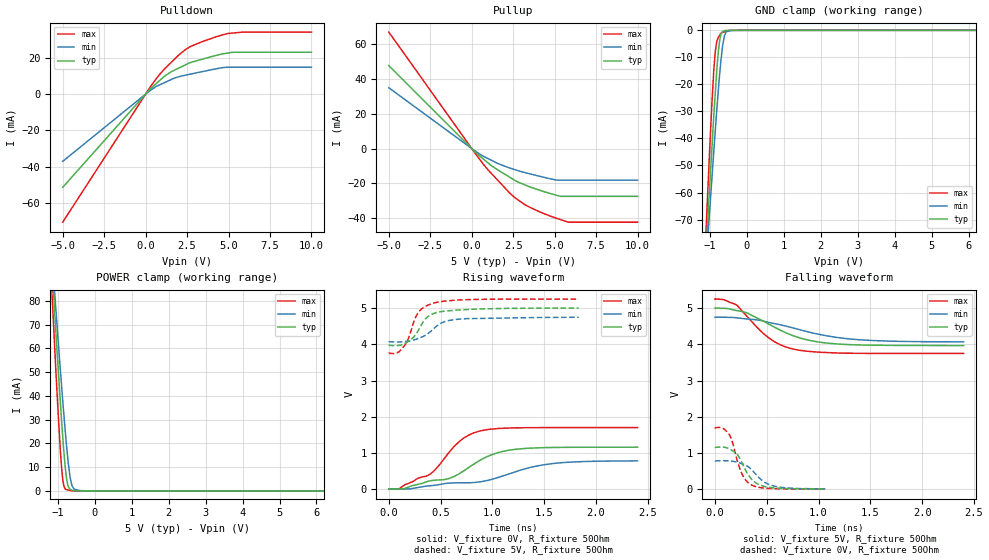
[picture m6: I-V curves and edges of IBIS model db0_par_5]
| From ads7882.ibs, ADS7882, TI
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|   db0_par_5 Model
[Model]   db0_par_5
Model_type   3-state
Polarity   Non-Inverting
Enable   Active-Low
Vmeas = 2.5
Vref = 2.5
Cref = 20pF
Rref = 50
|   typ   min   max
|   (nom PVT)   (Fast PVT)   (slow PVT)
|C_comp from frequency sweep method (F=1.5MHz)
|Average
C_comp   1.566e-12   1.438e-12   1.699e-12
|ON state : BUFFER OUTPUT TURNED HIGH
|C_comp   1.532e-12   1.413e-12   1.655e-12
|OFF state: BUFFER IN HIGH IMPEDANCE
|C_comp   1.600e-12   1.463e-12   1.743e-12
|C_comp from LC tank measurement(L=1nH)
|Resonant Frequency(Hz)   4.580e+09   4.690e+09   4.450e+09
|C_comp   1.209e-12   1.153e-12   1.280e-12
|ON state : BUFFER OUTPUT TURNED HIGH
|Resonant Frequency(Hz)   4.580e+09   4.690e+09   4.450e+09
|C_comp   1.209e-12   1.153e-12   1.280e-12
|OFF state: BUFFER IN HIGH IMPEDANCE
|Resonant Frequency   4.560e+09   4.660e+09   4.240e+09
|C_comp   1.219e-12   1.168e-12   1.410e-12
| Where nom  PVT is Nominal Process,  5V,  25C
|   Fast PVT is Strong Process,   5.25V,  -40C
|   Slow PVT is Weak Process,   4.75V,  85C
[Voltage Range]   5   4.75   5.25
|Ambient Temperature   25   85   -40
|Junction Temperature
[Temperature Range]   25   85   -40
[Pullup Reference]   5   4.75   5.25
[Pulldown Reference]   0   0   0
[Power Clamp Reference]   5   4.75   5.25
[GND Clamp Reference]   0   0   0
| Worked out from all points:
|   slope of the pulldown table from 0 to 0.75 V, typ, clamps not added: 112 ohm
|   slope of the pullup table from 0 to 0.75 V, typ, clamps not added: 117 ohm
|   GND clamp passes 1 mA (typ) near -0.69 V on its own axis
|   POWER clamp passes 1 mA (typ) near -0.68 V on its own axis
|   falling waveform, V_fixture 5V, R_fixture 50Ohm: 20-80 % time 464ps typ, 639ps min, 336ps max; typ from 5 V to 3.97 V
|   rising waveform, V_fixture 0V, R_fixture 50Ohm: 20-80 % time 569ps typ, 854ps min, 371ps max; typ from 0 V to 1.16 V
|   rising waveform, V_fixture 5V, R_fixture 50Ohm: 20-80 % time 161ps typ, 206ps min, 136ps max; typ from 3.97 V to 5 V
|   falling waveform, V_fixture 0V, R_fixture 50Ohm: 20-80 % time 145ps typ, 180ps min, 114ps max; typ from 1.16 V to 0.004 V
[Pulldown]
|   Voltage   I(typ)   I(min)   I(max)
-5V       -51.35mA   -37.04mA   -70.55mA
318.2mV   3.219mA    2.221mA    4.503mA
633.5mV   5.779mA    4.219mA    8.394mA
922mV     8.122mA    5.435mA    11.67mA
1.355V    11.23mA    7.258mA    15.81mA
1.988V    14.31mA    9.542mA    21.48mA
2.429V    16.27mA    10.51mA    24.74mA
2.712V    17.4mA     11.05mA    26.26mA
3.484V    19.42mA    12.52mA    29.14mA
4.965V    22.66mA    14.81mA    33.4mA
5.978V    23.1mA     14.81mA    34.19mA
10V       23.1mA     14.81mA    34.19mA
[GND Clamp]
|   Voltage   I(typ)   I(min)   I(max)
-5V       -1.068A    -890mA     -1.31A
-1.246V   -116.9mA   -115.3mA   -117.4mA
-1.029V   -63.34mA   -71.36mA   -51.02mA
-947mV    -43.94mA   -55.1mA    -27.49mA
-899.8mV  -32.81mA   -45.87mA   -16.01mA
-857.8mV  -23.89mA   -37.85mA   -8.451mA
-795mV    -11.49mA   -26.28mA   -3.385mA
-735mV    -3.698mA   -16.13mA   -1.807mA
-653.8mV  -426.8uA   -5.489mA   -770uA
-595mV    -58.31uA   -1.691mA   -511.2uA
-387.7mV  -38uA      -640.8nA   -2.42uA
10V       0A         0A         0A
[Pullup]
|   Voltage   I(typ)   I(min)   I(max)
-5V       47.68mA    34.91mA    66.91mA
60mV      -623.4uA   -448.2uA   -841.7uA
706.7mV   -6.059mA   -4.467mA   -9.092mA
1.355V    -10.95mA   -7.581mA   -16.06mA
2.271V    -16.38mA   -11.12mA   -25.4mA
2.639V    -18.53mA   -12.25mA   -28.49mA
3.485V    -21.99mA   -14.5mA    -33.71mA
5.175V    -27.03mA   -18.18mA   -40.29mA
5.81V     -27.49mA   -18.18mA   -42.31mA
10V       -27.49mA   -18.18mA   -42.34mA
[POWER Clamp]
|   Voltage   I(typ)   I(min)   I(max)
-5V       1.113A     944.2mA    1.331A
-1.246V   117.9mA    119mA      111.9mA
-1.047V   66.5mA     76.01mA    49.94mA
-983.8mV  50.92mA    62.67mA    31.7mA
-894.5mV  29.52mA    44.33mA    9.897mA
-857.8mV  21.62mA    36.97mA    4.223mA
-784.3mV  8.454mA    23.22mA    661.5uA
-715mV    1.908mA    11.99mA    397.4uA
-663.3mV  719.5uA    5.699mA    200uA
-615.8mV  353.6uA    2.348mA    18.88uA
-373.5mV  121.6uA    14.94uA    361.6nA
10V       0A         0A         0A
[Ramp]
R_load = 50
|   typ   min   max
dV/dt_r   0.694847/5.6865e-10   0.468119/8.54028e-10   1.0199/3.68733e-10
dV/dt_f   0.619077/4.64468e-10   0.408244/6.38188e-10   0.900192/3.36385e-10
[Falling Waveform]
V_fixture = 5V
V_fixture_min = 4.75V
V_fixture_max = 5.25V
R_fixture = 50Ohm
|   Time   V(typ)   V(min)   V(max)
0s        5V         4.75V      5.25V
77.81ps   4.997V     4.75V      5.24V
201.7ps   4.939V     4.737V     5.098V
318.7ps   4.859V     4.701V     4.745V
533.9ps   4.538V     4.597V     4.15V
629.9ps   4.394V     4.541V     3.991V
773.9ps   4.221V     4.439V     3.859V
1.003ns   4.065V     4.278V     3.786V
1.352ns   3.989V     4.137V     3.755V
2.4ns     3.968V     4.07V      3.75V
[Rising Waveform]
V_fixture = 0V
V_fixture_min = 0V
V_fixture_max = 0V
R_fixture = 50Ohm
|   Time   V(typ)   V(min)   V(max)
0s        3.943nV    8.547nV    3.686nV
99.94ps   2.181mV    87.9uV     16.86mV
404.1ps   231.6mV    94.94mV    424.9mV
575.7ps   289.3mV    162.9mV    994.2mV
677.9ps   423.4mV    175.5mV    1.311V
869.9ps   779.4mV    196.3mV    1.599V
1.099ns   1.041V     363.7mV    1.68V
1.496ns   1.146V     672.9mV    1.699V
1.88ns    1.156V     761.7mV    1.699V
2.4ns     1.158V     780.2mV    1.7V
[Rising Waveform]
V_fixture = 5V
V_fixture_min = 4.75V
V_fixture_max = 5.25V
R_fixture = 50Ohm
|   Time   V(typ)   V(min)   V(max)
0s        3.968V     4.068V     3.75V
77.81ps   3.965V     4.066V     3.763V
122.3ps   3.987V     4.067V     3.861V
177.1ps   4.06V      4.079V     4.086V
278ps     4.353V     4.156V     4.851V
356.9ps   4.714V     4.255V     5.056V
438.5ps   4.857V     4.445V     5.143V
543.4ps   4.915V     4.63V      5.194V
696.4ps   4.952V     4.699V     5.227V
1.832ns   4.999V     4.748V     5.25V
[Falling Waveform]
V_fixture = 0V
V_fixture_min = 0V
V_fixture_max = 0V
R_fixture = 50Ohm
|   Time   V(typ)   V(min)   V(max)
0s        1.158V     782.8mV    1.7V
77.81ps   1.162V     788.2mV    1.681V
140.7ps   1.113V     782.5mV    1.5V
166.4ps   1.069V     773.2mV    1.321V
206ps     989.7mV    750.7mV    889.4mV
261ps     732.3mV    701.6mV    422.7mV
356.7ps   266.6mV    531.2mV    111mV
458.7ps   90.45mV    232.7mV    35.95mV
576.9ps   32.84mV    81.56mV    14.8mV
1.064ns   3.876mV    7.478mV    752.7uV
